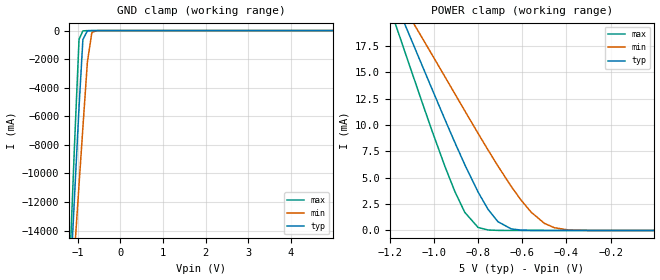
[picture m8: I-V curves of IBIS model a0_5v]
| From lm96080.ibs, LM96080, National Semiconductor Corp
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[Model] a0_5v
Model_type Input
Vinh = 2.0V
Vinl = 0.8V
C_comp   2.30pF   2.02pF   2.64pF
[Voltage Range]   5.0V   4.5V   5.5V
[Temperature Range]   25.0   125.0   -40.0
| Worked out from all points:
|   GND clamp passes 1 mA (typ) near -0.62 V on its own axis
|   POWER clamp passes 1 mA (typ) near -0.72 V on its own axis
[GND Clamp]
-5V       -243.4A    -190.1A    -303.1A
-1.175V   -17.86A    -20.28A    -15.88A
-1.07V    -11.55A    -15.5A     -7.894A
-965mV    -5.346A    -10.77A    -610.3mA
-875mV    -625mA     -6.781A    -21.36mA
-770mV    -21.11mA   -2.214A    -2.318mA
-665mV    -1.716mA   -131.7mA   -165.9uA
-560mV    -117.6uA   -9.782mA   -5.857uA
4.99V     1.052nA    0A         1.042nA
[POWER Clamp]
-5V       99.2mA     81.26mA    113.1mA
-1.205V   23.22mA    23.61mA    21.52mA
-1.16V    21mA       22.06mA    18.75mA
-1.115V   18.76mA    20.48mA    15.97mA
-1.055V   15.76mA    18.36mA    12.29mA
-905mV    8.357mA    12.98mA    3.701mA
-860mV    6.248mA    11.36mA    1.72mA
-800mV    3.652mA    9.224mA    289.5uA
-710mV    832.2uA    6.118mA    8.384uA
-605mV    34.52uA    2.871mA    217.7nA
-500mV    1.106uA    677.9uA    6.126nA
-5mV      1.056nA    9.899nA    1.156nA
